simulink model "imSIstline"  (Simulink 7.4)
settings: Solver=ode45  StartTime=0.0  StopTime=1.5  MaxStep=1e-3  RelTol=1e-3

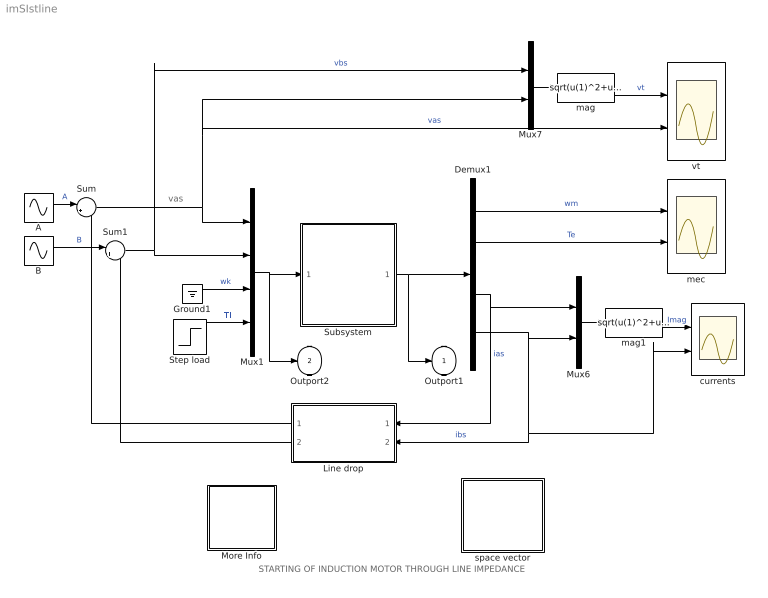
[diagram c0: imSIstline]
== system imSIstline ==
  note: vas
  note: STARTING OF INDUCTION MOTOR THROUGH LINE IMPEDANCE
  A : Sin  Amplitude=220*sqrt(2/3)  Bias=0  Frequency=2*pi*60  Phase=pi/2  Samples=10  SampleTime=0
  B : Sin  Amplitude=220*sqrt(2/3)  Bias=0  Frequency=2*pi*60  Phase=0  Samples=10  SampleTime=0
  Demux1 : Demux
  Ground1 : Ground
  Line drop : Subsystem  mask{Rline=0.01, Lline=0.8*0.001}
      mask prompts: Rline "Rline [ Ohms]"; Lline "Lline [H]"
  More Info : Subsystem
  Mux1 : Mux
  Mux6 : Mux  Inputs=2
  Mux7 : Mux  Inputs=2
  Step load : Step  Time=1.0  Before=0.0  After=10  SampleTime=0
  Subsystem : Subsystem  mask{Rs=0.531, Rr=0.408, L_param=[2.5 2.5 85]*0.001, wo=2*pi*60, J=0.1, p=4, ic=[0 0 0 0 0]}
      mask prompts: Rs "Stator resistance [Ohms]"; Rr "Rotor resistance [Ohms]"; L_param "Inductances Lsl,Lrl,Lm [H]"; wo "Base frequency [rad/s]"; J "Inertia  [kg.m^2]"; p "Number of poles"; ic "Initial conditions"
  Sum : Sum  Inputs=|+-  OutDataType=sfix(16)  OutScaling=2^0
  Sum1 : Sum  Inputs=|+-  OutDataType=sfix(16)  OutScaling=2^0
  currents : Scope  NumInputPorts=2
  mag : Fcn  Expr=sqrt(u(1)^2+u(2)^2)
  mag1 : Fcn  Expr=sqrt(u(1)^2+u(2)^2)
  mec : Scope  NumInputPorts=2
  space vector : Subsystem
  vt : Scope  NumInputPorts=2
  Outport1 : Outport
  Outport2 : Outport  Port=2
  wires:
  Demux1/1 -> mec/1  "wm"
  Demux1/2 -> mec/2  "Te"
  Ground1/1 -> Mux1/3  "wk"
  Step load/1 -> Mux1/4  "Tl"
  B/1 -> Sum1/1  "B"
  A/1 -> Sum/1  "A"
  mag/1 -> vt/1  "vt"
  Sum/1 -> Mux1/1, vt/2, Mux7/2  "vas"
  Sum1/1 -> Mux1/2, Mux7/1  "vbs"
  Mux7/1 -> mag/1
  Mux6/1 -> mag1/1
  mag1/1 -> currents/1  "Imag"
  Line drop/1(Outa) -> Sum/2
  Line drop/2(Outb) -> Sum1/2
  Demux1/3 -> Mux6/1, Line drop/1(Ina)  "ias"
  Demux1/4 -> Mux6/2, Line drop/2(Inb), currents/2  "ibs"
  Subsystem/1(Out) -> Demux1/1, Outport1/1
  Mux1/1 -> Subsystem/1(In), Outport2/1

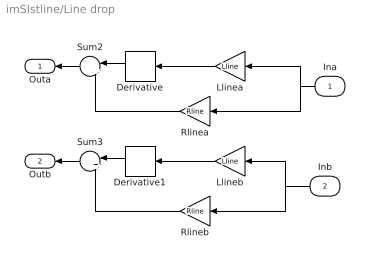
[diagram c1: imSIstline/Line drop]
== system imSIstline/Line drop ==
  Ina : Inport  OutDataType=sfix(16)  OutScaling=2^0
  Inb : Inport  Port=2  OutDataType=sfix(16)  OutScaling=2^0
  Derivative : Derivative
  Derivative1 : Derivative
  Llinea : Gain  Gain=Lline  ParameterDataType=sfix(16)  ParameterScaling=2^0  OutDataType=sfix(16)  OutScaling=2^0
  Llineb : Gain  Gain=Lline  ParameterDataType=sfix(16)  ParameterScaling=2^0  OutDataType=sfix(16)  OutScaling=2^0
  Rlinea : Gain  Gain=Rline  ParameterDataType=sfix(16)  ParameterScaling=2^0  OutDataType=sfix(16)  OutScaling=2^0
  Rlineb : Gain  Gain=Rline  ParameterDataType=sfix(16)  ParameterScaling=2^0  OutDataType=sfix(16)  OutScaling=2^0
  Sum2 : Sum  Inputs=|++  OutDataType=sfix(16)  OutScaling=2^0
  Sum3 : Sum  Inputs=|++  OutDataType=sfix(16)  OutScaling=2^0
  Outa : Outport
  Outb : Outport  Port=2
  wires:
  Llinea/1 -> Derivative/1
  Llineb/1 -> Derivative1/1
  Derivative/1 -> Sum2/1
  Rlinea/1 -> Sum2/2
  Rlineb/1 -> Sum3/2
  Derivative1/1 -> Sum3/1
  Sum2/1 -> Outa/1
  Sum3/1 -> Outb/1
  Ina/1 -> Llinea/1, Rlinea/1
  Inb/1 -> Llineb/1, Rlineb/1

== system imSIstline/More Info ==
  note: This demo simulates the starting characteristics of an induction motor including line impedance (voltage dip) [SI units] The induction machine is represented by an S_function.

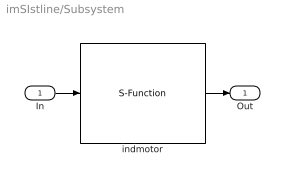
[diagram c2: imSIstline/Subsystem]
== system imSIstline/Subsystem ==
  In : Inport  OutDataType=sfix(16)  OutScaling=2^0
  indmotor : S-Function  FunctionName=immodSI  Parameters=Rs,Rr,L_param,J,p,wo,ic  EnableBusSupport=off
  Out : Outport
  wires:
  indmotor/1 -> Out/1
  In/1 -> indmotor/1

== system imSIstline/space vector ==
